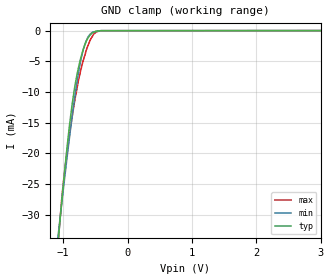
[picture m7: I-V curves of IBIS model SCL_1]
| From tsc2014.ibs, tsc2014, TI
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|   1.8V SCL Model
[Model] SCL_1
Model_type Input
Vinl = 0.54
Vinh = 1.26
|   typ   min   max
C_comp   3.1256960e-12   3.0017270e-12   3.3008290e-12
|Where nom PVT is NOM Process, 1.8V,27C
|   Fast PVT is Strong Process, 2.07V, -40C
|   Slow PVT is Weak Process, 1.53V, 85C
[Model Spec]
Vinl   0.54   0.459   0.621
Vinh   1.26   1.071   1.449
|VINL  0.3 DVDD, VINH  0.7 DVDD
[Voltage Range]   1.8   1.53   2.07
[Temperature Range]   27   85   -40
[Power Clamp Reference]   1.8   1.53   2.07
[GND Clamp Reference]   0   0   0
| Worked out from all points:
|   GND clamp passes 1 mA (typ) near -0.60 V on its own axis
[GND Clamp]
|   Voltage   I(typ)   I(min)   I(max)
-1.8V     -127mA     -105mA     -167.2mA
-1.074V   -33.84mA   -32.94mA   -34.16mA
-1.063V   -32.58mA   -31.94mA   -32.61mA
-985mV    -23.73mA   -24.76mA   -23.6mA
-896.4mV  -14.94mA   -16.98mA   -16.57mA
-816mV    -8.925mA   -10.58mA   -11.15mA
-754.3mV  -5.676mA   -6.39mA    -7.719mA
-686.9mV  -3.019mA   -3.062mA   -4.848mA
-616.8mV  -1.271mA   -1.109mA   -2.509mA
-538mV    -324.3uA   -229.6uA   -785.4uA
-410.4mV  -14.45uA   -11uA      -20.8uA
3.6V      0A         0A         0A
[POWER Clamp]
|   SCR cell used for ESD function. Effects occurr above VDD x 2
|   Voltage   I(typ)   I(min)   I(max)
-1.8V     0A         0A         0A
0V        0A         0A         0A
3.6V      0A         0A         0A
